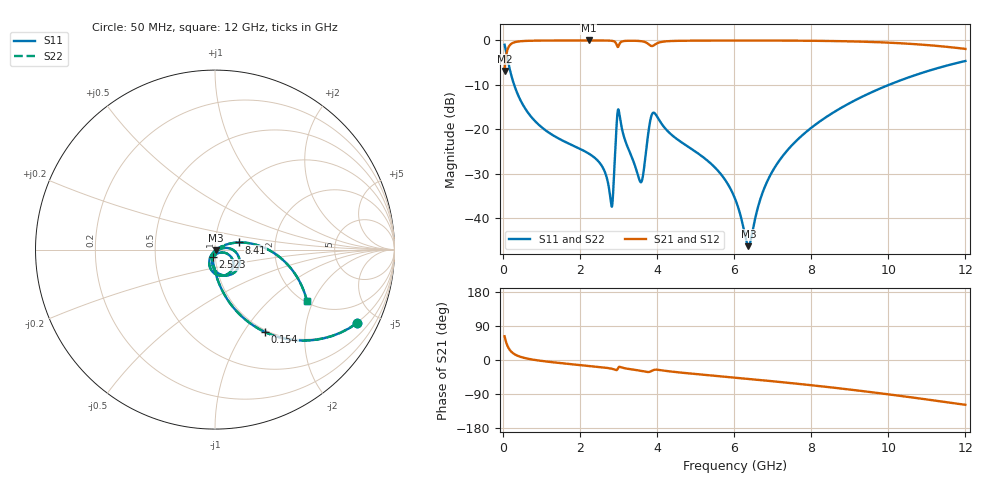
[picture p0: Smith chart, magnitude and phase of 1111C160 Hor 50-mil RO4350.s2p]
# GHz S MA R 50
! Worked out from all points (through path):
!   11951 points, 50 MHz to 12 GHz, reference 50 ohm
!   highest |S21| = -0.03 dB at 2.236 GHz (marker M1); lowest = -6.9 dB at 50 MHz (marker M2)
!   group delay of S21, straight-line fit = 28.6 ps
!   lowest |S11| = -46.3 dB at 6.373 GHz (marker M3), VSWR 1.01, Z = 50.3 - j0.376 ohm
!   |S11| at or under -10 dB: 297.1 MHz to 10.02 GHz (9.72 GHz wide, 188 % of centre)
!   |S22| runs from -46.3 to -1.0 dB; largest |S21 - S12| = 0
!   S11 on the Smith chart (normalised r, x): 50 MHz: 0.97, -3.87; 154 MHz: 0.97, -1.26; 2.523 GHz: 0.98, -0.08; 8.41 GHz: 1.30, +0.11; 12 GHz: 2.06, -1.78
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0.05  0.8912 -27.4  0.4535 62.6  0.4535 62.6  0.8912 -27.4
0.154  0.5385 -58.7  0.8422 31.3  0.8422 31.3  0.5385 -58.7
0.329  0.2887 -75.9  0.9568 14.0  0.9568 14.0  0.2887 -75.9
0.757  0.1354 -88.2  0.9899 1.4  0.9899 1.4  0.1354 -88.2
2.042  0.05921 -102.1  0.9966 -13.6  0.9966 -13.6  0.05921 -102.1
2.236  0.05326 -103.6  0.9966 -15.5  0.9966 -15.5  0.05326 -103.6
2.523  0.0416 -104.8  0.9963 -18.6  0.9963 -18.6  0.0416 -104.8
2.824  0.01365 -55.4  0.9883 -22.9  0.9883 -22.9  0.01365 -55.4
2.871  0.02193 -1.8  0.9795 -24.2  0.9795 -24.2  0.02193 -1.8
2.962  0.1264 -11.0  0.8774 -26.4  0.8774 -26.4  0.1264 -11.0
3.016  0.1584 -65.9  0.8864 -18.2  0.8864 -18.2  0.1584 -65.9
3.586  0.02541 -61.6  0.9784 -28.6  0.9784 -28.6  0.02541 -61.6
3.85  0.1385 -43.2  0.8647 -29.6  0.8647 -29.6  0.1385 -43.2
4.034  0.1325 -91.5  0.9377 -26.0  0.9377 -26.0  0.1325 -91.5
5.528  0.03637 -123.7  0.9938 -41.9  0.9938 -41.9  0.03637 -123.7
6.025  0.01665 -119.5  0.9947 -46.6  0.9947 -46.6  0.01665 -119.5
6.373  0.004863 -50.2  0.9948 -49.9  0.9948 -49.9  0.004863 -50.2
6.96  0.03164 25.3  0.9942 -55.7  0.9942 -55.7  0.03164 25.3
8.017  0.1052 20.3  0.9886 -66.7  0.9886 -66.7  0.1052 20.3
8.41  0.1391 16.6  0.9841 -71.1  0.9841 -71.1  0.1391 16.6
10.009  0.3152 -1.9  0.9416 -90.6  0.9416 -90.6  0.3152 -1.9
12  0.5859 -29.1  0.8012 -118.3  0.8012 -118.3  0.5859 -29.1
